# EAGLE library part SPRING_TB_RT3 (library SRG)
Spring Loaded Terminal Block 4UCON 0.10 pitch right angle 2 amps 20-26 AWG Adafruit: P/N 1074 Terminal block comes with 3 terminals, but the are modular so you can add or remove terminals
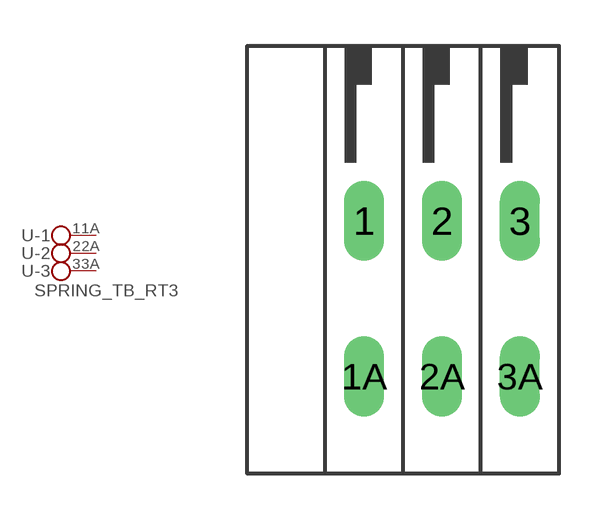
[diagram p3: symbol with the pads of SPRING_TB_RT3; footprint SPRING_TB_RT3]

Designator prefix -; gates -1=KL2 -2=KL2 -3=KL2V

## SPRING_TB_RT3  [SPRING_TB_RT3]
1  -1:1  pas
1A  -1:2  pas
2  -2:1  pas
2A  -2:2  pas
3  -3:1  pas
3A  -3:2  pas

## Footprint SPRING_TB_RT3 (pad centres in mm)
Spring Loaded Terminal Block 4UCON 0.10 pitch right angle 2 amps 20-26 AWG Adafruit: P/N 1074 Terminal block comes with 3 terminals, but the are modular so you can add or remove terminals
drill 0.8 long: 1 -2.54,2.54; 1A -2.54,-2.54; 2 0,2.54; 2A 0,-2.54; 3 2.54,2.54; 3A 2.54,-2.54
